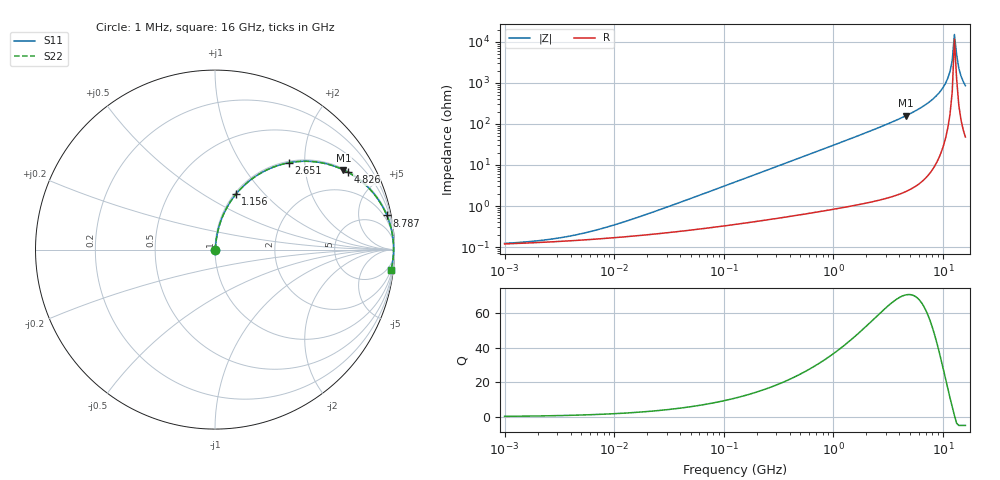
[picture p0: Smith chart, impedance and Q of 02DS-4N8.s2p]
# MHz S MA R 50
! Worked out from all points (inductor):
!   211 points, 1 MHz to 16 GHz, reference 50 ohm
!   read as one part in series: L = 4.8 nH near 20.01 MHz
!   highest Q = 70.4 at 4.609 GHz (marker M1), where L = 5.51 nH
!   self-resonance near 12.71 GHz
!   S11 on the Smith chart (normalised r, x): 1 MHz: 1.00, +0.00; 1.156 GHz: 1.02, +0.70; 2.651 GHz: 1.03, +1.67; 4.826 GHz: 1.05, +3.39; 8.787 GHz: 1, +10; 16 GHz: 2, -17
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1  0.001226 14.2  0.9988 -0.0  0.9988 -0.0  0.001226 14.2
2.51416  0.001524 29.7  0.9987 -0.0  0.9987 -0.0  0.001524 29.7
5.25662  0.002171 46.7  0.9985 -0.1  0.9985 -0.1  0.002171 46.7
26.3872  0.008223 74.5  0.9978 -0.5  0.9978 -0.5  0.008223 74.5
132.458  0.03994 82.6  0.9956 -2.3  0.9956 -2.3  0.03994 82.6
664.915  0.1959 76.7  0.9739 -11.3  0.9739 -11.3  0.1959 76.7
1156.12  0.3291 69.3  0.936 -19.2  0.936 -19.2  0.3291 69.3
1750.57  0.4699 60.8  0.8732 -28.0  0.8732 -28.0  0.4699 60.8
2650.66  0.6359 49.6  0.7612 -39.5  0.7612 -39.5  0.6359 49.6
3187.38  0.7102 43.9  0.693 -45.2  0.693 -45.2  0.7102 43.9
4608.83  0.8422 31.8  0.5274 -57.4  0.5274 -57.4  0.8422 31.8
4826.25  0.8562 30.3  0.5047 -58.9  0.5047 -58.9  0.8562 30.3
6664.19  0.9353 19.8  0.3394 -69.3  0.3394 -69.3  0.9353 19.8
8787.49  0.9762 11.2  0.195 -77.4  0.195 -77.4  0.9762 11.2
10566.8  0.9905 5.7  0.0994 -81.7  0.0994 -81.7  0.9905 5.7
11587.3  0.9939 3.0  0.0519 -81.8  0.0519 -81.8  0.9939 3.0
12134  0.9947 1.6  0.02835 -78.5  0.02835 -78.5  0.9947 1.6
12706.4  0.995 0.2  0.006544 -39.4  0.006544 -39.4  0.995 0.2
13305.8  0.9946 -1.1  0.02024 73.9  0.02024 73.9  0.9946 -1.1
13933.5  0.9936 -2.5  0.04363 80.3  0.04363 80.3  0.9936 -2.5
14590.9  0.992 -3.8  0.06727 81.3  0.06727 81.3  0.992 -3.8
16000  0.987 -6.6  0.1147 80.2  0.1147 80.2  0.987 -6.6
